| PCA9505 IBIS Model
[IBIS Ver]   3.2
[Comment Char]   |_char
| VDD: nom: 2.5v, min:2.2v, max: 2.8v
[File name]   pca9505_2_5.ibs
[File Rev]   1
[Date]   Aug 20, 2008 2:35:49 PM
[Source]
Generated by Seshadri Venkataramanan using IBIS Toolkit at NXP, Tempe
[Notes]
[Disclaimer]
(C) Copyright 2007 NXP Semiconductors
All rights reserved
NXP Semiconductors (NXP) does not warrant that this model and any other
accompanying information (Model) accurately or fully represents the
operating characteristics and specifications of the semiconductor
products to which the Model relates.  Moreover, the Model is furnished
on an "as is" and with "all faults" basis, and without support or
warranty of any kind.  NXP disclaims all warranties, whether expressed
or implied or statutory, including without limitation all implied
warranties of non-infringement, merchantability and fitness for any
purpose, and those arising from a course of dealing or usage of trade.
NXP does not convey any license under its or any third party's patents,
copyrights or other intellectual property or proprietary rights.
You and your company assume any and all risks and liability arising out
of the application or use of the Model.
In no event shall NXP be liable for any direct, indirect, special,
consequential or incidental damages, however caused, whether in
warranty, contract or tort (including negligence), strict liability or
other legal theory, including, without limitation, for lost profits,
business interruption, or corruption or loss of data or information,
arising out of or in connection with the use of or the inability to use
the Model, even if NXP has been advised of the possibility of such
damages.
NXP provides the Model as a courtesy to our customers. You and your
company shall not distribute, convey, sell, or give the Model to anyone
else without receiving prior written permission from NXP.
NXP reserves the right to make changes without notice to the Model to
improve reliability, function, or design.
Please be aware that your receipt and subsequent use of the Model shall
serve as acceptance of these terms and conditions.  If you do not
accept these terms, return or destroy the Model immediately.
[Copyright]
2008
| tssop56
[Component]   PCA9505DGG
Si_location Pin
Timing_location Pin
[Manufacturer]   NXP Semiconductors
[Package]
R_pkg   75.2m   58.5m   91.8m
L_pkg   5.35n   3.09n   7.61n
C_pkg   0.809p   0.429p   1.189p
[Package Model]   tssop56
[Pin] signal_name   model_name   R_pin   L_pin   C_pin
1   SDA   SDAIO   83.3mO   7.61nH   1.008pF
2   SCL   SCL   84.3mO   7.08nH   1.189pF
3   IO0_0   IO   85.6mO   6.49nH   1.083pF
4   IO0_1   IO   86.7mO   5.96nH   0.966pF
5   IO0_2   IO   89.2mO   5.38nH   0.868pF
6   VSS   GND   91.4mO   4.93nH   0.821pF
7   IO0_3   IO   87.3mO   4.50nH   0.757pF
8   IO0_4   IO   91.8mO   4.27nH   0.707pF
9   IO0_5   IO   80.8mO   3.91nH   0.652pF
10   IO0_6   IO   72.3mO   3.69nH   0.635pF
11   VSS   GND   65.9mO   3.46nH   0.623pF
12   IO0_7   IO   62.8mO   3.30nH   0.590pF
13   IO1_0   IO   60.3mO   3.15nH   0.554pF
14   IO1_1   IO   58.5mO   3.09nH   0.541pF
15   IO1_2   IO   58.5mO   3.09nH   0.429pF
16   IO1_3   IO   60.3mO   3.15nH   0.432pF
17   IO1_4   IO   62.8mO   3.30nH   0.565pF
18   VDD   POWER   65.9mO   3.46nH   0.603pF
19   IO_5   IO   72.3mO   3.69nH   0.639pF
20   IO_6   IO   80.8mO   3.91nH   0.642pF
21   IO_7   IO   91.8mO   4.27nH   0.669pF
22   IO2_0   IO   87.3mO   4.50nH   0.730pF
23   VSS   GND   91.4mO   4.93nH   0.787pF
24   IO2_1   IO   89.2mO   5.38nH   0.861pF
25   IO2_2   IO   86.7mO   5.96nH   0.922pF
26   IO2_3   IO   85.6mO   6.49nH   1.014pF
27   A0   ADDR   84.3mO   7.08nH   1.141pF
28   A1   ADDR   83.3mO   7.61nH   1.268pF
29   A2   ADDR   83.3mO   7.61nH   1.310pF
30   Oeb   RESETb   84.3mO   7.08nH   1.189pF
31   IO2_4   IO   85.6mO   6.49nH   1.083pF
32   IO2_5   IO   86.7mO   5.96nH   0.966pF
33   IO2_6   IO   89.2mO   5.38nH   0.868pF
34   VSS   GND   91.4mO   4.93nH   0.821pF
35   IO2_7   IO   87.3mO   4.50nH   0.757pF
36   IO3_0   IO   91.8mO   4.27nH   0.707pF
37   IO3_1   IO   80.8mO   3.91nH   0.652pF
38   IO3_2   IO   72.3mO   3.69nH   0.635pF
39   VSS   GND   65.9mO   3.46nH   0.623pF
40   IO3_3   IO   62.8mO   3.30nH   0.590pF
41   IO3_4   IO   60.3mO   3.15nH   0.554pF
42   IO3_5   IO   58.5mO   3.09nH   0.541pF
43   IO3_6   IO   58.5mO   3.09nH   0.429pF
44   IO3_7   IO   60.3mO   3.15nH   0.432pF
45   IO4_0   IO   62.8mO   3.30nH   0.565pF
46   VDD   POWER   65.9mO   3.46nH   0.603pF
47   IO4_1   IO   72.3mO   3.69nH   0.639pF
48   IO4_2   IO   80.8mO   3.91nH   0.642pF
49   IO4_3   IO   91.8mO   4.27nH   0.669pF
50   IO4_4   IO   87.3mO   4.50nH   0.730pF
51   VSS   GND   91.4mO   4.93nH   0.787pF
52   IO4_5   IO   89.2mO   5.38nH   0.861pF
53   IO4_6   IO   86.7mO   5.96nH   0.922pF
54   IO4_7   IO   85.6mO   6.49nH   1.014pF
55   INTb   INT_OUT   84.3mO   7.08nH   1.141pF
56   RESETb   RESETb   83.3mO   7.61nH   1.268pF
| tssop56
[Component]   PCA9506DGG
Si_location Pin
Timing_location Pin
[Manufacturer]   NXP Semiconductors
[Package]
R_pkg   75.2m   58.5m   91.8m
L_pkg   5.35n   3.09n   7.61n
C_pkg   0.809p   0.429p   1.189p
[Package Model]   tssop56
[Pin] signal_name   model_name   R_pin   L_pin   C_pin
1   SDA   SDAIO   83.3mO   7.61nH   1.008pF
2   SCL   SCL   84.3mO   7.08nH   1.189pF
3   IO0_0   IO   85.6mO   6.49nH   1.083pF
4   IO0_1   IO   86.7mO   5.96nH   0.966pF
5   IO0_2   IO   89.2mO   5.38nH   0.868pF
6   VSS   GND   91.4mO   4.93nH   0.821pF
7   IO0_3   IO   87.3mO   4.50nH   0.757pF
8   IO0_4   IO   91.8mO   4.27nH   0.707pF
9   IO0_5   IO   80.8mO   3.91nH   0.652pF
10   IO0_6   IO   72.3mO   3.69nH   0.635pF
11   VSS   GND   65.9mO   3.46nH   0.623pF
12   IO0_7   IO   62.8mO   3.30nH   0.590pF
13   IO1_0   IO   60.3mO   3.15nH   0.554pF
14   IO1_1   IO   58.5mO   3.09nH   0.541pF
15   IO1_2   IO   58.5mO   3.09nH   0.429pF
16   IO1_3   IO   60.3mO   3.15nH   0.432pF
17   IO1_4   IO   62.8mO   3.30nH   0.565pF
18   VDD   POWER   65.9mO   3.46nH   0.603pF
19   IO_5   IO   72.3mO   3.69nH   0.639pF
20   IO_6   IO   80.8mO   3.91nH   0.642pF
21   IO_7   IO   91.8mO   4.27nH   0.669pF
22   IO2_0   IO   87.3mO   4.50nH   0.730pF
23   VSS   GND   91.4mO   4.93nH   0.787pF
24   IO2_1   IO   89.2mO   5.38nH   0.861pF
25   IO2_2   IO   86.7mO   5.96nH   0.922pF
26   IO2_3   IO   85.6mO   6.49nH   1.014pF
27   A0   ADDR   84.3mO   7.08nH   1.141pF
28   A1   ADDR   83.3mO   7.61nH   1.268pF
29   A2   ADDR   83.3mO   7.61nH   1.310pF
30   Oeb   RESETb   84.3mO   7.08nH   1.189pF
31   IO2_4   IO   85.6mO   6.49nH   1.083pF
32   IO2_5   IO   86.7mO   5.96nH   0.966pF
33   IO2_6   IO   89.2mO   5.38nH   0.868pF
34   VSS   GND   91.4mO   4.93nH   0.821pF
35   IO2_7   IO   87.3mO   4.50nH   0.757pF
36   IO3_0   IO   91.8mO   4.27nH   0.707pF
37   IO3_1   IO   80.8mO   3.91nH   0.652pF
38   IO3_2   IO   72.3mO   3.69nH   0.635pF
39   VSS   GND   65.9mO   3.46nH   0.623pF
40   IO3_3   IO   62.8mO   3.30nH   0.590pF
41   IO3_4   IO   60.3mO   3.15nH   0.554pF
42   IO3_5   IO   58.5mO   3.09nH   0.541pF
43   IO3_6   IO   58.5mO   3.09nH   0.429pF
44   IO3_7   IO   60.3mO   3.15nH   0.432pF
45   IO4_0   IO   62.8mO   3.30nH   0.565pF
46   VDD   POWER   65.9mO   3.46nH   0.603pF
47   IO4_1   IO   72.3mO   3.69nH   0.639pF
48   IO4_2   IO   80.8mO   3.91nH   0.642pF
49   IO4_3   IO   91.8mO   4.27nH   0.669pF
50   IO4_4   IO   87.3mO   4.50nH   0.730pF
51   VSS   GND   91.4mO   4.93nH   0.787pF
52   IO4_5   IO   89.2mO   5.38nH   0.861pF
53   IO4_6   IO   86.7mO   5.96nH   0.922pF
54   IO4_7   IO   85.6mO   6.49nH   1.014pF
55   INTb   INT_OUT   84.3mO   7.08nH   1.141pF
56   RESETb   RESETb   83.3mO   7.61nH   1.268pF
[Define Package Model]  tssop56
[Manufacturer]   Unknown
[OEM]   Unknown
[Description]   none
[Number Of Pins]   56
[Pin Numbers]
   1   |   1 =
   2   |   2 =
   3   |   3 =
   4   |   4 =
   5   |   5 =
   6   |   6 =
   7   |   7 =
   8   |   8 =
   9   |   9 =
  10   |  10 =
  11   |  11 =
  12   |  12 =
  13   |  13 =
  14   |  14 =
  15   |  15 =
  16   |  16 =
  17   |  17 =
  18   |  18 =
  19   |  19 =
  20   |  20 =
  21   |  21 =
  22   |  22 =
  23   |  23 =
  24   |  24 =
  25   |  25 =
  26   |  26 =
  27   |  27 =
  28   |  28 =
  29   |  29 =
  30   |  30 =
  31   |  31 =
  32   |  32 =
  33   |  33 =
  34   |  34 =
  35   |  35 =
  36   |  36 =
  37   |  37 =
  38   |  38 =
  39   |  39 =
  40   |  40 =
  41   |  41 =
  42   |  42 =
  43   |  43 =
  44   |  44 =
  45   |  45 =
  46   |  46 =
  47   |  47 =
  48   |  48 =
  49   |  49 =
  50   |  50 =
  51   |  51 =
  52   |  52 =
  53   |  53 =
  54   |  54 =
  55   |  55 =
  56   |  56 =
[Model Data]
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[End Model Data]
[End Package Model]
[Define Package Model]  HVQFN56
[Manufacturer]  ST-NXP Wireless
|[Simulated] Chris Hunat
|[Approved] Wayne Nunn, Roger Real
[OEM]  Unknown
[Description]  Full package model
[Number Of Pins]  56
[Pin Numbers]
|Pin Num   Terminal Name
1   | lead1:pin1
2   | lead2:pin2
3   | lead3:pin3
4   | lead4:pin4
5   | lead5:pin5
6   | lead6:pin6
7   | lead7:pin7
8   | lead8:pin8
9   | lead9:pin9
10   | lead10:pin10
11   | lead11:pin11
12   | lead12:pin12
13   | lead13:pin13
14   | lead14:pin14
15   | lead15:pin15
16   | lead16:pin16
17   | lead17:pin17
18   | lead18:pin18
19   | lead19:pin19
20   | lead20:pin20
21   | lead21:pin21
22   | lead22:pin22
23   | lead23:pin23
24   | lead24:pin24
25   | lead25:pin25
26   | lead26:pin26
27   | lead27:pin27
28   | lead28:pin28
29   | lead29:pin29
30   | lead30:pin30
31   | lead31:pin31
32   | lead32:pin32
33   | lead33:pin33
34   | lead34:pin34
35   | lead35:pin35
36   | lead36:pin36
37   | lead37:pin37
38   | lead38:pin38
39   | lead39:pin39
40   | lead40:pin40
41   | lead41:pin41
42   | lead42:pin42
43   | lead43:pin43
44   | lead44:pin44
45   | lead45:pin45
46   | lead46:pin46
47   | lead47:pin47
48   | lead48:pin48
49   | lead49:pin49
50   | lead50:pin50
51   | lead51:pin51
52   | lead52:pin52
53   | lead53:pin53
54   | lead54:pin54
55   | lead55:pin55
56   | lead56:pin56
[Model Data]
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[End Model Data]
[End Package Model]
| Models and submodels in the file (6): ADDR (Input), SCL (Input), SDAIO (I/O_open_drain), RESETb (Input), INT_OUT (Open_drain), IO (I/O)
